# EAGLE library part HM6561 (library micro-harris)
MICROCONTROLLER/MEMORY DEVICE
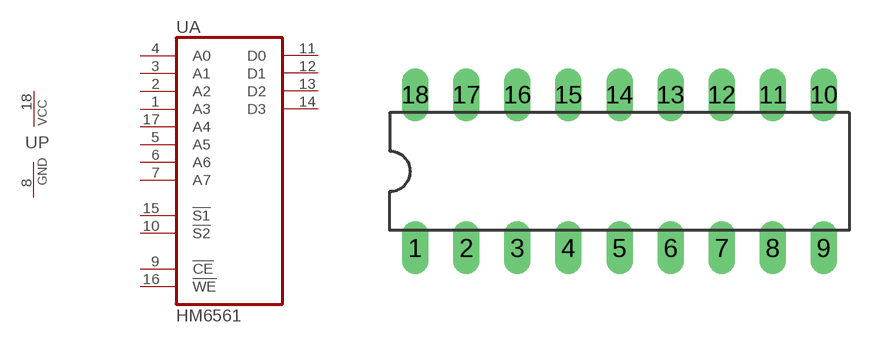
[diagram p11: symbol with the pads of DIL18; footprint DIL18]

Designator prefix U; gates A=HM6561 P=PWRN

## HM6561 (OC_FARNELL: unknown; OC_NEWARK: unknown)  [DIL18]
1  A:A3  in
2  A:A2  in
3  A:A1  in
4  A:A0  in
5  A:A5  in
6  A:A6  in
7  A:A7  in
8  P:GND  pwr
9  A:!CE  in
10  A:!S2  in
11  A:D0
12  A:D1
13  A:D2
14  A:D3
15  A:!S1  in
16  A:!WE  in
17  A:A4  in
18  P:VCC  pwr

## Footprint DIL18 (pad centres in mm)
Dual In Line Package
drill 0.813 long: 1 -10.16,-3.81; 2 -7.62,-3.81; 3 -5.08,-3.81; 4 -2.54,-3.81; 5 0,-3.81; 6 2.54,-3.81; 7 5.08,-3.81; 8 7.62,-3.81; 9 10.16,-3.81; 10 10.16,3.81; 11 7.62,3.81; 12 5.08,3.81; 13 2.54,3.81; 14 0,3.81; 15 -2.54,3.81; 16 -5.08,3.81; 17 -7.62,3.81; 18 -10.16,3.81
